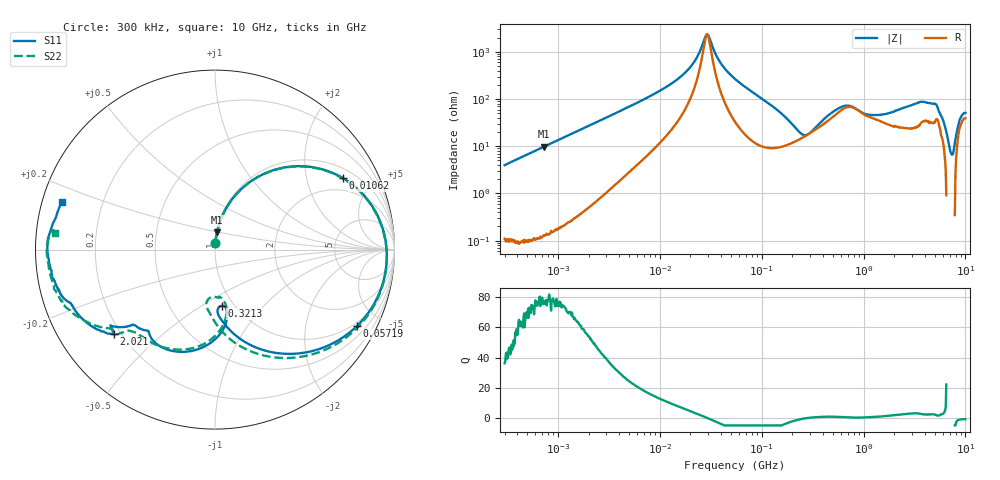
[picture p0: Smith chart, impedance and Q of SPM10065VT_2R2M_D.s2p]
! S-Parameter Data Generated by TDK Corporation
! Copyright(C) 2020 TDK Corporation.
! All Rights Reserved.
! TDK P/N: SPM10065VT-2R2M-D (Inductor)
! Property: L=2.2uH at 100kHz
! Size(LxWxT): 10.5x10x6.5mm
! Model Type: s2p (Touchstone File Format Version 1.0)
! Frequency: DC=Yes Start=0.3MHz Stop=10000MHz 802points Log-sweep
! Model Generated on Aug. 18, 2020
! Port Assignments:
!  1 ---@@@--- 2
! Applicable Conditions:
!  Temperature = 25 degC
!  DC Bias Current = 0 A
!  Small Signal Operation
! Terms and conditions regarding TDK Simulation Models
! (1)This simulation model is being provided solely for informational purposes. Please refer to the specifications of the products in terms of detailed characteristics of such products.
! (2)In no event shall TDK Corporation of any of its subsidiaries be liable for any loss or damage arising, directly or indirectly,
!  From any information contained in this simulation model, including, but not limited to loss or damages arising from any inaccuracies, omissions or errors in connection with such information.
! (3)Any and all copyrights on this simulation model are owned by TDK Corporation.
!  Duplication or redistribution of this simulation model without prior written permission from TDK Corporation is prohibited.
! (4)This simulation model is subject to any modification or change without any prior notice.
! (5)Neither TDK Corporation nor any of its subsidiaries shall make any warranty, express or implied,
!  Including but not limited to the correctness, implied warranties of merchantability and fitness for a particular purpose with respect to this simulation models.
! (6)The use of this simulation model shall be deemed to have consented to the terms and conditions hereof.
# Hz S MA R 50
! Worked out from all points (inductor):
!   801 points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, 300 kHz to 10 GHz, reference 50 ohm
!   read as one part in series: L = 2.12 uH near 318.3 kHz
!   highest Q = 78.2 at 733.4 kHz (marker M1), where L = 2.14 uH
!   self-resonance near 29.19 MHz
!   S11 on the Smith chart (normalised r, x): 300 kHz: 1.00, +0.08; 10.62 MHz: 1.38, +3.32; 57.19 MHz: 0.86, -3.77; 321.3 MHz: 0.88, -0.61; 2.021 GHz: 0.17, -0.35; 10 GHz: 0.06, +0.15
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300000  0.03936 86.3  0.9983 -2.3  0.9979 -2.3  0.03883 86.0
733382  0.09674 83.6  0.9942 -5.7  0.9937 -5.7  0.09655 83.5
1713600  0.222 76.0  0.9712 -13.1  0.971 -13.1  0.222 75.9
3822232  0.4527 60.7  0.8771 -27.5  0.8769 -27.5  0.4527 60.6
9671944  0.7901 32.2  0.5552 -53.5  0.5551 -53.5  0.7904 31.9
1.062202e7  0.8175 29.1  0.5108 -56.2  0.5107 -56.2  0.8179 28.8
1.945436e7  0.9354 9.1  0.2101 -69.4  0.2101 -69.5  0.9357 8.5
2.90046e7  0.9586 -3.9  0.0409 -8.8  0.04088 -8.9  0.959 -4.8
3.955676e7  0.9477 -14.6  0.1609 60.6  0.1608 60.6  0.9481 -15.8
5.477226e7  0.9057 -26.7  0.3276 55.5  0.3275 55.5  0.9059 -28.5
5.718581e7  0.8975 -28.4  0.3498 54.2  0.3498 54.2  0.8977 -30.2
9.679373e7  0.7474 -50.6  0.604 33.0  0.6038 33.0  0.7462 -53.8
1.630679e8  0.5413 -72.0  0.765 6.7  0.7648 6.7  0.5337 -77.6
3.126428e8  0.32 -85.7  0.7345 -29.4  0.7343 -29.5  0.299 -99.1
3.212744e8  0.3149 -83.4  0.733 -30.4  0.7328 -30.4  0.2833 -98.3
4.388767e8  0.379 -79.8  0.6631 -51.8  0.6629 -51.8  0.2787 -81.4
5.911415e8  0.5023 -90.3  0.4848 -70.1  0.4847 -70.1  0.4138 -83.1
8.643532e8  0.6192 -117.7  0.3592 -74.6  0.3591 -74.6  0.5871 -108.4
1.767019e9  0.6673 -139.7  0.2494 -141.3  0.2494 -141.3  0.677 -137.7
2.020878e9  0.7337 -140.0  0.1883 -157.7  0.1883 -157.7  0.7249 -142.6
5.040844e9  0.9101 -168.5  0.01836 171.8  0.01834 171.5  0.9124 -164.2
1e10  0.8906 162.7  0.02105 140.6  0.02097 140.6  0.8987 174.2
